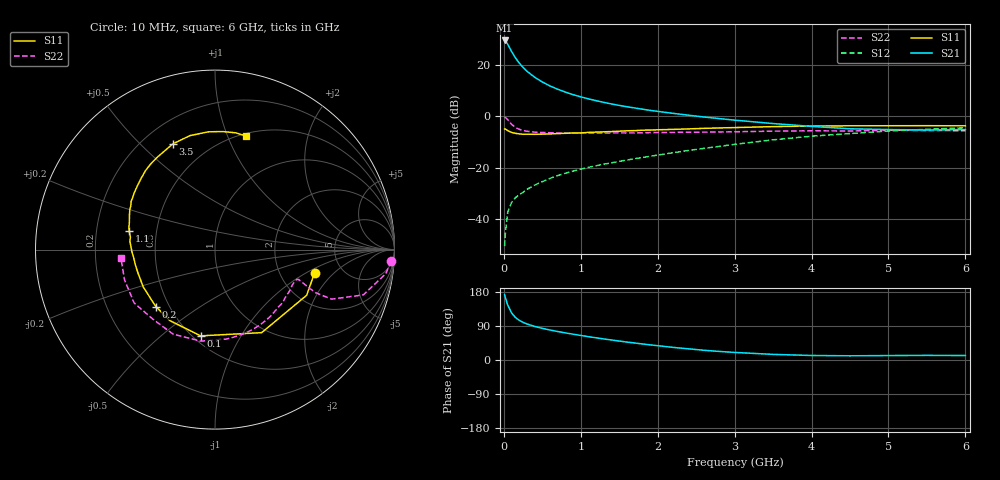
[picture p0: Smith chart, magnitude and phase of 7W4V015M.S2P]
! Infineon Technologies  Discrete & RF Semiconductors
! BFS17W
! Si NPN RF Bipolar Junction Transistor in SOT323
! VCE = 4 V  IC = 15 mA
! Common Emitter S-Parameters:  August  1999
# GHz  S  MA  R  50
!  f  S11  S21  S12  S22
! GHz  MAG  ANG  MAG  ANG  MAG  ANG  MAG  ANG
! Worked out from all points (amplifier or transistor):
!   36 points, 10 MHz to 6 GHz, reference 50 ohm
!   highest |S21| = 29.8 dB at 10 MHz (marker M1)
!   |S21| within 3 dB of that: start of sweep to 77.32 MHz
!   unconditionally stable (mu >= 1): 335.5 MHz to 2.301 GHz; 5.05 GHz to end of sweep
!   at 250 MHz: K = 0.91, MSG = 24.4 dB, |S12| = -29.7 dB
!   at 1.4 GHz: K = 1.18, MAG = 8.9 dB, |S12| = -18.1 dB
!   at 6 GHz: K = 1.06, MAG = -1.8 dB, |S12| = -4.4 dB
!   S11 on the Smith chart (normalised r, x): 10 MHz: 3.14, -1.21; 100 MHz: 0.55, -0.69; 200 MHz: 0.42, -0.34; 1.1 GHz: 0.35, +0.09; 3.5 GHz: 0.32, +0.63; 6 GHz: 0.52, +1.16
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0.01  0.5697 -13.2  30.76 172.4  0.0029 80.8  0.9825 -3.6
0.02  0.5705 -26.5  30.17 164.5  0.0052 83.5  0.9618 -8.0
0.05  0.5307 -60.7  25.98 145.1  0.0133 67.0  0.8634 -17.0
0.1  0.4872 -99.5  18.81 124.4  0.0208 58.8  0.7062 -23.0
0.15  0.4687 -122.3  14.1 112.3  0.0257 55.2  0.6111 -23.2
0.2  0.4575 -136.1  11.13 104.8  0.0295 57.7  0.5622 -22.1
0.25  0.4491 -145.9  9.11 99.3  0.0329 58.6  0.5314 -21.0
0.3  0.4505 -152.6  7.699 95.2  0.0374 60.1  0.5152 -20.4
0.4  0.4484 -162.7  5.871 88.6  0.0453 63.0  0.4943 -19.7
0.5  0.4516 -169.0  4.735 83.5  0.0531 65.2  0.4866 -19.9
0.6  0.4552 -174.2  3.956 79.1  0.0615 66.4  0.4809 -20.8
0.7  0.4629 -178.4  3.417 75.2  0.0698 67.7  0.4774 -22.1
0.9  0.4765 174.4  2.678 68.1  0.0853 68.7  0.4735 -25.5
1.1  0.4888 168.0  2.213 61.5  0.1013 69.4  0.4745 -29.7
1.3  0.5012 162.1  1.888 55.5  0.1167 69.7  0.4739 -34.6
1.6  0.5248 154.6  1.551 47.3  0.1402 70.2  0.4766 -42.1
2.2  0.5596 140.6  1.152 33.3  0.1954 70.7  0.489 -58.9
2.8  0.597 126.8  0.91 22.6  0.2602 68.4  0.4981 -77.0
3.5  0.634 111.8  0.728 14.8  0.3492 62.8  0.5163 -98.9
4.5  0.6571 93.3  0.575 11.1  0.4636 50.1  0.5197 -132.1
5.5  0.6607 80.0  0.545 12.2  0.5621 37.3  0.5316 -161.5
6  0.6563 74.9  0.555 11.8  0.6009 31.1  0.526 -174.6
